PROGRAM MAIN
VAR
	
	Listener: FB_EventListener;
END_VAR

Listener(
	SubscribeOption:= , 
	EventClassID:=  TC_EVENT_CLASSES.MyEvent, 
	bError=> , 
	hr=> , 
	nCntMessagesSent=> , 
	nCntAlarmsRaised=> , 
	nCntAlarmsConfirmed=> , 
	nCntAlarmsCleared=> , 
	sLastMessageText=> , 
	sLastAlarmText=> , 
	CurrentGUID=> , 
	Tips=> );

END_PROGRAM
